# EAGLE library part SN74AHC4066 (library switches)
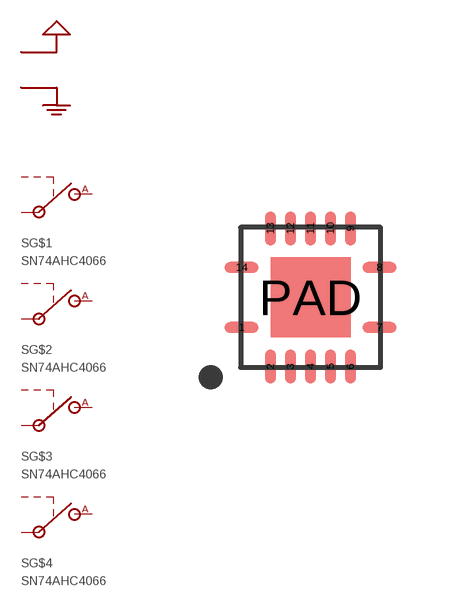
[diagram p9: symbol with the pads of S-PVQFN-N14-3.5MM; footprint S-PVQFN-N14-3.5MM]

Designator prefix S; gates G$1=SPST-DIGITAL G$2=SPST-DIGITAL G$3=SPST-DIGITAL G$4=SPST-DIGITAL G$5=PWR

## SN74AHC4066-RGY (DIGIKEY: 296-15258-1-ND)  [S-PVQFN-N14-3.5MM]
1  G$1:IN
2  G$1:A
3  G$2:A
4  G$2:IN
5  G$2:CTRL
6  G$3:CTRL
7  G$5:GND
8  G$3:IN
9  G$3:A
10  G$4:A
11  G$4:IN
12  G$4:CTRL
13  G$1:CTRL
14  G$5:VCC

## Footprint S-PVQFN-N14-3.5MM (pad centres in mm)
smd 0.85 x 0.28: 1 -1.725,-0.75; 7 1.725,-0.75; 8 1.725,0.75; 14 -1.725,0.75
smd 0.28 x 0.85: 2 -1,-1.725; 3 -0.5,-1.725; 4 0,-1.725; 5 0.5,-1.725; 6 1,-1.725; 9 1,1.725; 10 0.5,1.725; 11 0,1.725; 12 -0.5,1.725; 13 -1,1.725
smd 2 x 2: PAD 0,0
